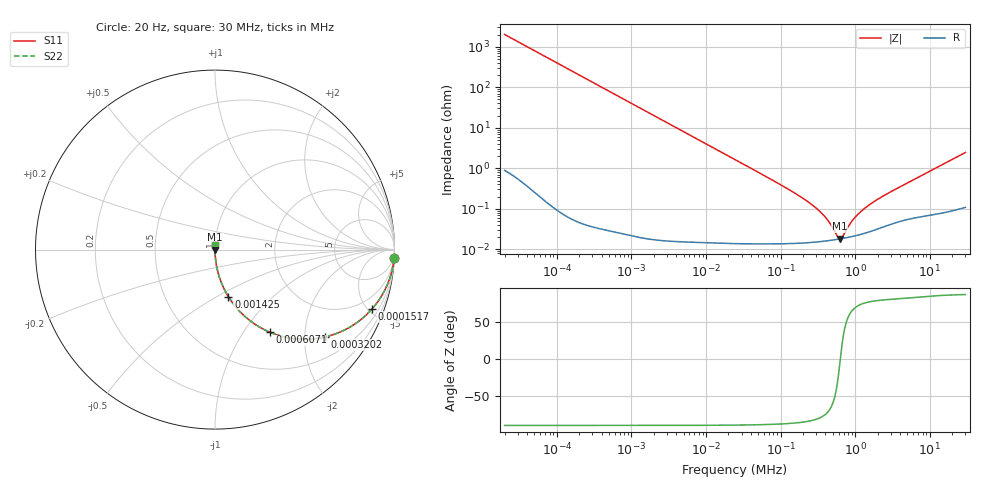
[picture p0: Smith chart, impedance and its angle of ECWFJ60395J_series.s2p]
!  *** S-Parameter ***
!  Copyright (C) Panasonic Industry
!  Plastic Film Capacitor (ECWFJ)
!  Parts No. ECWFJ60395J
!  Connection Mode : Series
!  1  o---||---o  2
!  GND o--------o GND
!  Conditions : Temperature = 20 ¡æ  DC Bias = 0 V
! Frequency Range : 20 Hz  -  30 MHz  [ 401 Steps ]
# Hz S RI R 50
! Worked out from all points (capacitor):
!   401 points, 20 Hz to 30 MHz, reference 50 ohm
!   read as one part in series: C = 3.95 uF near 21.47 Hz
!   lowest |Z| = 18.2 mohm at 622.5 kHz (marker M1)
!   series resonance near 631.9 kHz, so ESL is about 16 nH
!   S11 on the Smith chart (normalised r, x): 20 Hz: 1, -40; 151.7 Hz: 1.00, -5.31; 320.2 Hz: 1.00, -2.52; 607.1 Hz: 1.00, -1.33; 1.425 kHz: 1.00, -0.57; 30 MHz: 1.00, +0.05
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20  0.9975 -0.0495  0.00248 0.0495  0.00248 0.0495  0.9975 -0.0495
60.21117  0.9781 -0.1461  0.0219 0.1461  0.0219 0.1461  0.9781 -0.1461
151.748  0.8759 -0.3296  0.1241 0.3296  0.1241 0.3296  0.8759 -0.3296
216.5336  0.7761 -0.4167  0.2239 0.4167  0.2239 0.4167  0.7761 -0.4167
320.1605  0.6133 -0.4869  0.3867 0.4869  0.3867 0.4869  0.6133 -0.4869
607.1443  0.3062 -0.4607  0.6938 0.4607  0.6938 0.4607  0.3062 -0.4607
930.1964  0.1583 -0.3648  0.8417 0.3648  0.8417 0.3648  0.1583 -0.3648
1425.139  0.0743 -0.2619  0.9257 0.2619  0.9257 0.2619  0.0743 -0.2619
2344.34  0.0289 -0.167  0.9711 0.167  0.9711 0.167  0.0289 -0.167
6122.189  0.00447 -0.0656  0.9955 0.0656  0.9955 0.0656  0.00447 -0.0656
24494.9  0.000408 -0.0164  0.9996 0.0164  0.9996 0.0164  0.000408 -0.0164
121307  0.000148 -0.0032  0.9999 0.0032  0.9999 0.0032  0.000148 -0.0032
265198.4  0.00015 -0.00124  0.9999 0.00124  0.9999 0.00124  0.00015 -0.00124
406306.4  0.000161 -0.000573  0.9998 0.000573  0.9998 0.000573  0.000161 -0.000573
579770.3  0.000177 -0.000107  0.9998 0.000107  0.9998 0.000107  0.000177 -0.000107
622495.7  0.000181 -1.85e-05  0.9998 1.85e-05  0.9998 1.85e-05  0.000181 -1.85e-05
668369.8  0.000185 6.97e-05  0.9998 -6.97e-05  0.9998 -6.97e-05  0.000185 6.97e-05
888257.1  0.000205 0.000427  0.9998 -0.000427  0.9998 -0.000427  0.000205 0.000427
1180485  0.000233 0.000811  0.9998 -0.000811  0.9998 -0.000811  0.000233 0.000811
1684468  0.000286 0.00137  0.9997 -0.00137  0.9997 -0.00137  0.000286 0.00137
2871218  0.000408 0.00249  0.9996 -0.00249  0.9996 -0.00249  0.000408 0.00249
3e7  0.00169 0.0245  0.9983 -0.0245  0.9983 -0.0245  0.00169 0.0245
